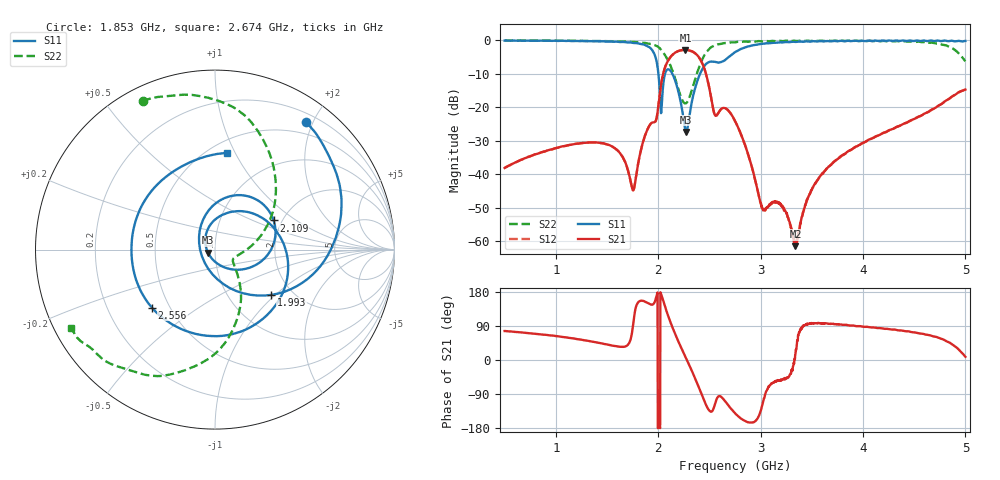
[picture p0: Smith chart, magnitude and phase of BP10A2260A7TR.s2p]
!Agilent Technologies,E8358A,US41080443,A.07.50.56
!Agilent E8358A: A.07.50.56
!Date: Tuesday, December 16, 2014 13:56:09
!Correction: S11(Full 2 Port(1,2))
!S21(Full 2 Port(1,2))
!S12(Full 2 Port(1,2))
!S22(Full 2 Port(1,2))
!S2P File: Measurements: S11, S21, S12, S22:
# Hz S  dB  R 50
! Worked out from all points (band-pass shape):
!   1601 points, 500 MHz to 5 GHz, reference 50 ohm
!   highest |S21| = -2.84 dB at 2.266 GHz (marker M1); lowest = -61.5 dB at 3.341 GHz (marker M2)
!   |S21| within 3 dB of the highest: 2.101 GHz to 2.414 GHz (313.3 MHz wide, 13.9 % of centre)
!   lowest |S11| = -27.4 dB at 2.275 GHz (marker M3), VSWR 1.09, Z = 46.2 - j1.59 ohm
!   |S11| at or under -10 dB: 2.002 GHz to 2.066 GHz (64.37 MHz wide, 3.16 % of centre); 2.139 GHz to 2.408 GHz (269.7 MHz wide, 11.9 % of centre)
!   |S22| runs from -18.9 to 0.0 dB; largest |S21 - S12| = 0.0039
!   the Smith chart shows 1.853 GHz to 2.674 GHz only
!   S11 on the Smith chart (normalised r, x): 1.853 GHz: 0.32, +1.90; 1.993 GHz: 1.57, -0.95; 2.109 GHz: 1.81, +0.68; 2.556 GHz: 0.40, -0.33; 2.674 GHz: 0.61, +0.93
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5e8  -0.08 164.5  -38.12 76.5  -38.16 76.6  -0.05 172.9
1.250938e9  -0.18 132.8  -30.68 53.5  -30.73 53.6  -0.14 156.1
1.59125e9  -0.37 104.3  -32.53 36.2  -32.58 36.3  -0.28 140.8
1.754375e9  -0.76 79.2  -44.81 92.0  -44.82 92.0  -0.46 127.7
1.852812e9  -1.20 54.5  -30.23 156.1  -30.30 156.2  -0.73 116.1
1.94e9  -2.86 13.8  -24.59 145.9  -24.58 146.2  -1.15 99.9
1.993438e9  -7.89 -38.7  -21.50 178.2  -21.52 178.5  -1.81 85.0
2.001875e9  -9.93 -52.2  -19.46 -177.4  -19.45 -177.3  -1.98 82.1
2.10875e9  -8.76 26.4  -5.44 107.7  -5.48 107.8  -6.79 42.3
2.26625e9  -26.92 -130.6  -2.84 8.0  -2.87 8.0  -18.85 -28.2
2.274688e9  -27.37 -156.3  -2.85 3.1  -2.88 3.1  -18.73 -30.9
2.373125e9  -12.99 68.4  -4.18 -56.6  -4.19 -56.5  -10.37 -61.4
2.4575e9  -7.37 -18.8  -9.05 -112.8  -9.09 -112.9  -4.12 -95.1
2.555938e9  -6.42 -137.5  -22.42 -114.7  -22.47 -114.5  -1.50 -128.9
2.674062e9  -5.31 83.2  -20.61 -115.7  -20.70 -115.8  -0.80 -151.5
2.75e9  -3.52 24.1  -24.06 -140.7  -24.11 -140.3  -0.60 -160.6
2.98625e9  -1.14 -62.0  -46.85 -145.7  -46.92 -146.0  -0.21 -178.6
3.340625e9  -0.46 -110.0  -61.50 15.6  -60.91 19.0  -0.18 166.5
3.500938e9  -0.28 -121.6  -44.49 97.3  -44.54 96.5  -0.16 162.7
4.251875e9  -0.04 -153.8  -26.90 81.7  -26.96 81.7  -0.24 145.4
4.822812e9  -0.20 -168.6  -17.81 48.5  -17.84 48.6  -1.64 101.7
5e9  -0.17 -171.3  -14.70 8.4  -14.78 8.2  -6.25 17.2
